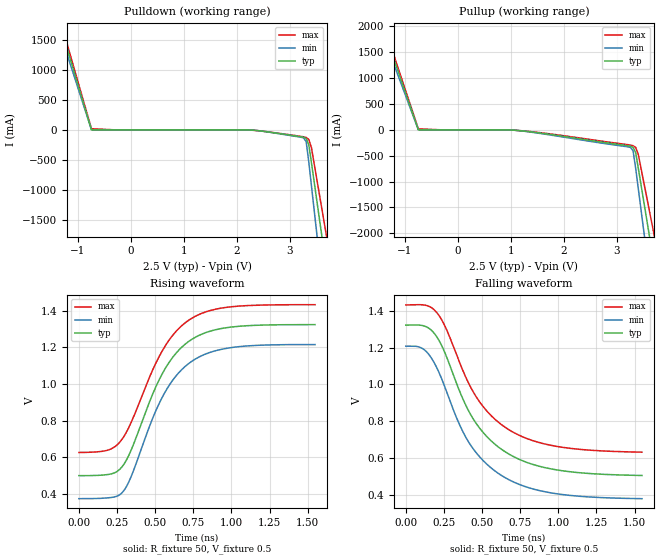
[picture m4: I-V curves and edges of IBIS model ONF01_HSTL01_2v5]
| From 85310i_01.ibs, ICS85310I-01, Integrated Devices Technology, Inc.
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[Model]   ONF01_HSTL01_2v5
Model_type   Output_ECL
Polarity   Non-Inverting
|   typ   min   max
C_comp   2pF   1.5pF   2.5pF
Vmeas = 0.825V
Rref = 50
Cref = 0
Vref = 0.5V
|   typ   min   max
[Voltage range]   2.5V   2.375V   2.625V
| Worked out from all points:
|   rising waveform, R_fixture 50, V_fixture 0.5: 20-80 % time 273ps typ, 275ps min, 280ps max; typ from 0.5 V to 1.32 V
|   falling waveform, R_fixture 50, V_fixture 0.5: 20-80 % time 331ps typ, 332ps min, 330ps max; typ from 1.32 V to 0.504 V
[Pulldown]
|Voltage   I (typ)   I (min)   I (max)
-2.5V     6.581A     7.946A     5.777A
-1.62V    3.059A     3.451A     2.841A
-1.18V    1.303A     1.209A     1.377A
-740mV    1.386mA    169.5uA    18.55mA
2.274V    -4.057mA   -2.715mA   -5.464mA
3.31V     -144.6mA   -197.8mA   -127.9mA
3.359V    -248.5mA   -537.3mA   -160.2mA
3.408V    -548.5mA   -928.9mA   -295.5mA
3.507V    -1.163A    -1.712A    -808.4mA
3.606V    -1.778A    -2.495A    -1.321A
3.704V    -2.392A    -3.278A    -1.834A
5V        -10.47A    -13.57A    -8.575A
[Pullup]
|Voltage   I (typ)   I (min)   I (max)
-2.5V     6.581A     7.946A     5.777A
-1.62V    3.059A     3.451A     2.841A
-1.18V    1.303A     1.209A     1.377A
-740mV    1.386mA    169.5uA    18.55mA
1.14V     -13mA      -13.73mA   -11.95mA
3.31V     -336.9mA   -402.8mA   -305.8mA
3.408V    -741.1mA   -1.134A    -473.9mA
3.507V    -1.356A    -1.917A    -987.3mA
3.556V    -1.663A    -2.308A    -1.244A
3.606V    -1.971A    -2.7A      -1.501A
3.704V    -2.585A    -3.483A    -2.014A
5V        -10.66A    -13.77A    -8.757A
[Ramp]
|   typ   min   max
dV/dt_r   0.658/0.426n   0.672/0.43n   0.644/0.437n
dV/dt_f   0.655/0.544n   0.664/0.546n   0.642/0.541n
R_load =   50.0000
[Rising Waveform]
R_fixture = 50
V_fixture = 0.5   | VCC_typ - 2V
V_fixture_max = 0.625   | VCC_max - 2V
V_fixture_min = 0.375   | VCC_min - 2V
C_fixture = 0.0p
| Time   typ   min   max
0s        500.4mV    375mV      627mV
193.9ps   507mV      379.7mV    640.8mV
290.1ps   556.6mV    414mV      707.7mV
341.3ps   637.1mV    492.9mV    788.2mV
473.2ps   924.1mV    791.2mV    1.057V
549.2ps   1.06V      931.9mV    1.185V
639.2ps   1.17V      1.047V     1.289V
740.1ps   1.243V     1.124V     1.358V
1.009ns   1.311V     1.2V       1.422V
1.548ns   1.324V     1.215V     1.433V
[Falling Waveform]
R_fixture = 50
V_fixture = 0.5   | VCC_typ - 2V
V_fixture_max = 0.625   | VCC_max - 2V
V_fixture_min = 0.375   | VCC_min - 2V
C_fixture = 0.0p
| Time   typ   min   max
0s        1.322V     1.208V     1.432V
117.9ps   1.319V     1.19V      1.432V
206.4ps   1.255V     1.085V     1.388V
266.9ps   1.151V     962.5mV    1.299V
406.5ps   864.5mV    693.5mV    1.016V
502.7ps   742.5mV    589mV      883.8mV
622.2ps   649.6mV    506.8mV    784mV
769.6ps   582.7mV    447.3mV    713.1mV
954.2ps   539.4mV    408.8mV    667.7mV
1.548ns   503.8mV    377.5mV    630.7mV
